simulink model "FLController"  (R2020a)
settings: Solver=VariableStepAuto  StartTime=0.0  StopTime=20  RelTol=1e-3
InitFcn:
  | initParams
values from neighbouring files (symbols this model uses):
  K1 = 5    [initParams.m]
  K2 = 10    [initParams.m]
  K3 = 10    [initParams.m]
  x0 = [0.2;0.1]    [initParams.m]

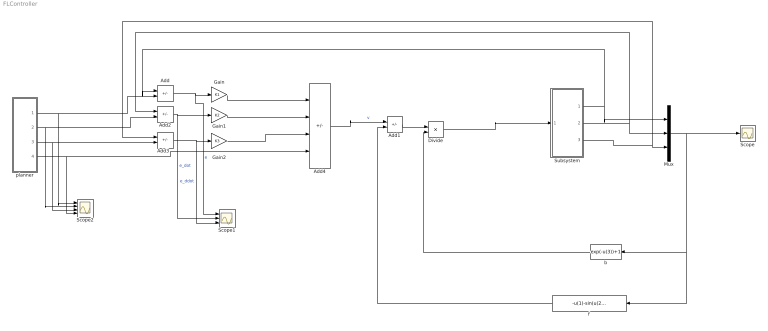
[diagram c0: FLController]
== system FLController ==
  Add{,1..3} (4 alike) : Sum  Inputs=+-
  Add4 : Sum  Inputs=---+
  Divide : Product  Inputs=*/
  Gain : Gain  Gain=K1
  Gain1 : Gain  Gain=K2
  Gain2 : Gain  Gain=K3
  Mux : Mux  Inputs=3
  Scope : Scope
  Scope1 : Scope  NumInputPorts=3
  Scope2 : Scope  NumInputPorts=4
  Subsystem : Subsystem
  b : Fcn  Expr=exp(-u(3))+1
  f : Fcn  Expr=-u(1)-sin(u(2))
  planner : Subsystem
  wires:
  Subsystem/1(x1) -> Add/1, Mux/1
  Subsystem/2(x2) -> Mux/2, Add2/1
  Subsystem/3(x3) -> Add3/1, Mux/3
  Mux/1 -> Scope/1, b/1, f/1
  f/1 -> Add1/2
  Add1/1 -> Divide/1
  b/1 -> Divide/2
  Divide/1 -> Subsystem/1(u)
  planner/1(xd) -> Scope2/1, Add/2
  planner/2(xd_dot) -> Scope2/2, Add2/2
  planner/3(xd_ddot) -> Scope2/3, Add3/2
  Add/1 -> Scope1/1, Gain/1  "e"
  Add2/1 -> Scope1/2, Gain1/1  "e_dot"
  Add3/1 -> Scope1/3, Gain2/1  "e_ddot"
  Add4/1 -> Add1/1  "v"
  Gain/1 -> Add4/1
  Gain1/1 -> Add4/2
  Gain2/1 -> Add4/3
  planner/4(xd_dddot) -> Scope2/4, Add4/4

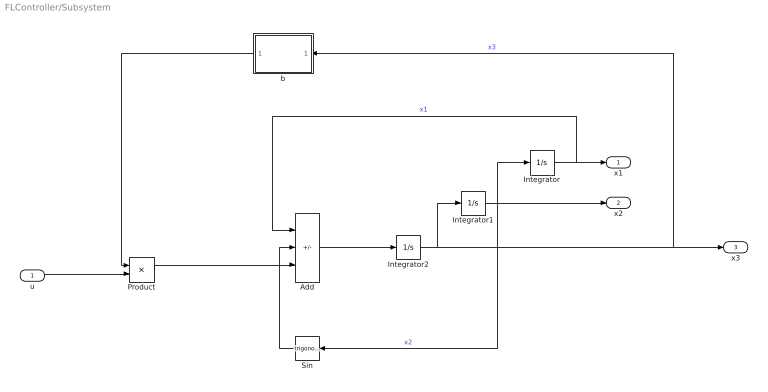
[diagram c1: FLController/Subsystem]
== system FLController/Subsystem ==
  u : Inport
  Add : Sum  Inputs=--+
  Integrator : Integrator  InitialCondition=x0(1)
  Integrator1 : Integrator  InitialCondition=x0(2)
  Integrator2 : Integrator  InitialCondition=x0(3)
  Product : Product
  Sin : Trigonometry
  b : MATLAB Function  TreatAsAtomicUnit=on
  x1 : Outport
  x2 : Outport  Port=2
  x3 : Outport  Port=3
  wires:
  Integrator/1 -> Add/1, x1/1  "x1"
  Sin/1 -> Add/2
  Integrator1/1 -> x2/1, Sin/1, Integrator/1  "x2"
  u/1 -> Product/2
  Integrator2/1 -> b/1(x3), x3/1, Integrator1/1  "x3"
  Add/1 -> Integrator2/1
  Product/1 -> Add/3
  b/1(y) -> Product/1

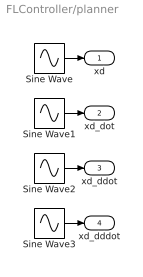
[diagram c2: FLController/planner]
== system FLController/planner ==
  Sine Wave : Sin  SampleTime=0
  Sine Wave1 : Sin  Phase=pi/2  SampleTime=0
  Sine Wave2 : Sin  Amplitude=-1  SampleTime=0
  Sine Wave3 : Sin  Amplitude=-1  Phase=pi/2  SampleTime=0
  xd : Outport
  xd_dot : Outport  Port=2
  xd_ddot : Outport  Port=3
  xd_dddot : Outport  Port=4
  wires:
  Sine Wave1/1 -> xd_dot/1
  Sine Wave2/1 -> xd_ddot/1
  Sine Wave3/1 -> xd_dddot/1
  Sine Wave/1 -> xd/1

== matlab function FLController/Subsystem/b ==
function y = fcn(x3)

y = exp(-x3)+1;
